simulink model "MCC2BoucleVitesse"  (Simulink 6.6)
settings: Solver=ode45  StartTime=0.0  StopTime=0.4  RelTol=1e-3
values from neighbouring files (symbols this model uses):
  Cr = Cmax/4    (= 0.0068445)    [moteur.m]
  h = 50e-6    (= 5e-05)    [moteur.m]
  J = 2e-6    (= 2e-06)    [moteur.m]
  K = 0.0234    [moteur.m]
  Kiv1 = 1.414/Te/K*(K*K+R*kv)    (= 320.291794118)    [moteur.m]
  Kpv1 = Kiv1*Tem2    (= 2.43542533937)    [moteur.m]
  kv = 13e-6    (= 1.3e-05)    [moteur.m]
  L = 0.000238    [moteur.m]
  omegaref = 300    [moteur.m]
  R = 2.19    [moteur.m]
libraries: simulink x1

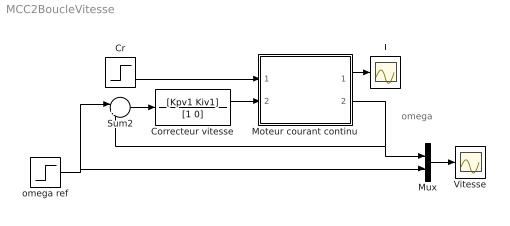
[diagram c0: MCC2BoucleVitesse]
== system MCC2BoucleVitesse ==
  note: omega
  Correcteur vitesse : TransferFcn  Numerator=[Kpv1 Kiv1]  Denominator=[1 0]
  Cr : Step  Time=0.25  After=Cr  SampleTime=0
  I : Scope
  Moteur courant continu : Subsystem
  Mux : Mux  Inputs=2
  Sum2 : Sum  Inputs=|+-
  Vitesse : Scope
  omega ref : Step  Time=0.05  After=omegaref  SampleTime=0
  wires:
  omega ref/1 -> Mux/2, Sum2/1
  Correcteur vitesse/1 -> Moteur courant continu/2(Uref)
  Mux/1 -> Vitesse/1
  Sum2/1 -> Correcteur vitesse/1
  Cr/1 -> Moteur courant continu/1(Cr)
  Moteur courant continu/1(I) -> I/1
  Moteur courant continu/2(omega) -> Sum2/2, Mux/1

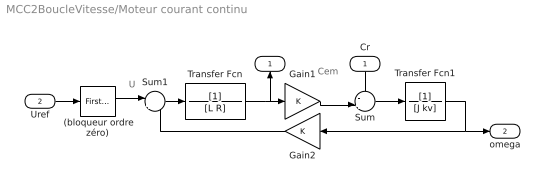
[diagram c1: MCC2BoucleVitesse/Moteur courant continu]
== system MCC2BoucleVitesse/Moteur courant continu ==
  note: U
  note: I
  note: Cem
  Cr : Inport  Orientation=down
  Uref : Inport  Port=2
  " (bloqueur ordre zéro)" : simulink/Discrete/First-Order Hold  SystemSampleTime=-1  Ts=h
  Gain1 : Gain  Gain=K
  Gain2 : Gain  Orientation=left  Gain=K
  Sum : Sum  Inputs=-+|
  Sum1 : Sum  Inputs=|+-
  Transfer Fcn : TransferFcn  Denominator=[L R]
  Transfer Fcn1 : TransferFcn  Denominator=[J kv]
  I : Outport  Orientation=up
  omega : Outport  Port=2
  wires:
  Transfer Fcn/1 -> Gain1/1, I/1
  Gain1/1 -> Sum/2
  Sum/1 -> Transfer Fcn1/1
  Transfer Fcn1/1 -> Gain2/1, omega/1
  " (bloqueur ordre zéro)"/1 -> Sum1/1
  Sum1/1 -> Transfer Fcn/1
  Gain2/1 -> Sum1/2
  Cr/1 -> Sum/1
  Uref/1 -> " (bloqueur ordre zéro)"/1
